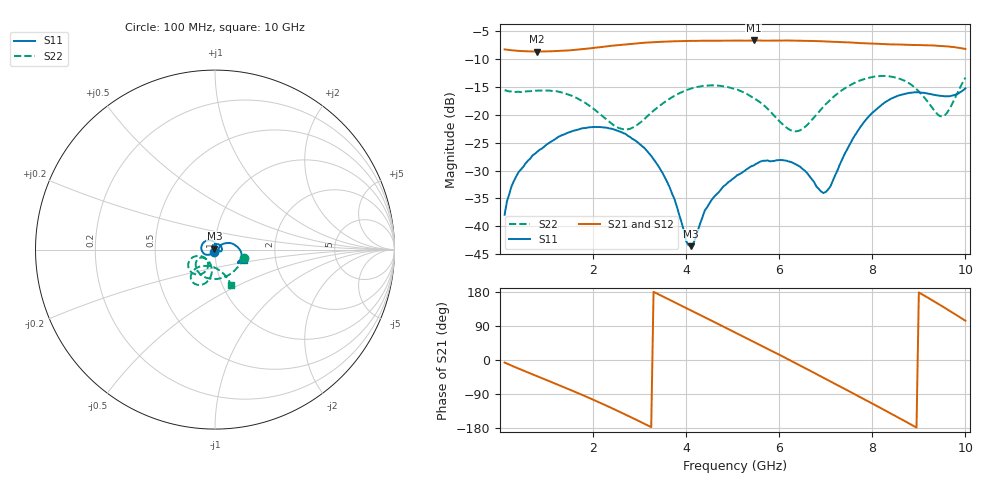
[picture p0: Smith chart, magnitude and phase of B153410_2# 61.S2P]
!  2-Port S-parameters saved by WinCal
! VAR MeasName=S-Parameters (CALIBRATED_DATA) read from VNA (N5245A)
! VAR MeasDate=2016-12-23 10:02:39
! VAR NAME=B153410_2# 61
! VAR FILENAME=B153410_2# 61.S2P
! VAR DATE=2016-12-23 10:02:39
! VAR PHYS_PORTS=1,2
# Hz S DB R 50
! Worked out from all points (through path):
!   199 points, 100 MHz to 10 GHz, reference 50 ohm
!   highest |S21| = -6.73 dB at 5.45 GHz (marker M1); lowest = -8.7 dB at 800 MHz (marker M2)
!   group delay of S21, straight-line fit = 171 ps
!   lowest |S11| = -43.5 dB at 4.1 GHz (marker M3), VSWR 1.01, Z = 49.7 + j0.6 ohm
!   |S11| at or under -10 dB: start of sweep to end of sweep
!   |S22| runs from -23.0 to -13.1 dB; largest |S21 - S12| = 0.0035
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1e8  -37.92 -102.7  -8.33 -6.7  -8.33 -6.7  -15.62 -16.1
3e8  -31.86 -123.2  -8.53 -17.5  -8.55 -17.5  -15.96 -39.9
8e8  -26.66 -141.6  -8.72 -42.9  -8.71 -42.8  -15.70 -87.8
1.75e9  -22.49 -178.2  -8.31 -91.2  -8.30 -91.2  -17.49 -143.6
2.25e9  -22.30 156.6  -7.83 -118.3  -7.84 -118.4  -20.60 -151.1
2.7e9  -23.46 130.5  -7.43 -144.3  -7.43 -144.3  -22.69 -133.1
3.4e9  -29.14 89.2  -7.01 173.8  -7.01 173.8  -18.61 -112.1
3.75e9  -35.11 73.9  -6.88 152.4  -6.88 152.5  -16.63 -116.8
4e9  -42.61 89.3  -6.82 137.1  -6.83 137.2  -15.64 -122.6
4.1e9  -43.53 115.0  -6.82 131.0  -6.81 131.1  -15.36 -125.2
4.4e9  -37.16 143.9  -6.78 112.7  -6.78 112.7  -14.82 -133.7
5.05e9  -31.20 94.3  -6.75 72.8  -6.76 73.0  -15.41 -151.4
5.45e9  -29.10 54.8  -6.73 48.3  -6.75 48.3  -17.04 -159.4
6.25e9  -28.46 -6.8  -6.75 -1.8  -6.77 -1.8  -22.81 -140.0
6.7e9  -31.50 -19.4  -6.82 -30.7  -6.83 -30.6  -20.95 -104.9
6.95e9  -34.03 -1.1  -6.89 -46.8  -6.91 -46.7  -18.58 -98.5
7.05e9  -33.40 12.8  -6.93 -53.4  -6.95 -53.2  -17.73 -98.0
7.7e9  -22.76 29.8  -7.17 -95.4  -7.19 -95.2  -14.00 -107.3
8.35e9  -17.42 1.8  -7.42 -137.9  -7.43 -137.6  -13.13 -123.8
8.95e9  -16.01 -22.4  -7.54 -178.4  -7.54 -178.1  -15.44 -135.6
9.5e9  -16.66 -29.8  -7.74 141.9  -7.74 142.2  -20.35 -102.2
1e10  -15.30 -18.9  -8.26 103.7  -8.29 103.9  -13.38 -65.4
